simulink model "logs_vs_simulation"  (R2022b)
settings: Solver=FixedStepAuto  StartTime=0.0  StopTime=29  FixedStep=0.001  RelTol=1e-3
libraries: vrlib x2

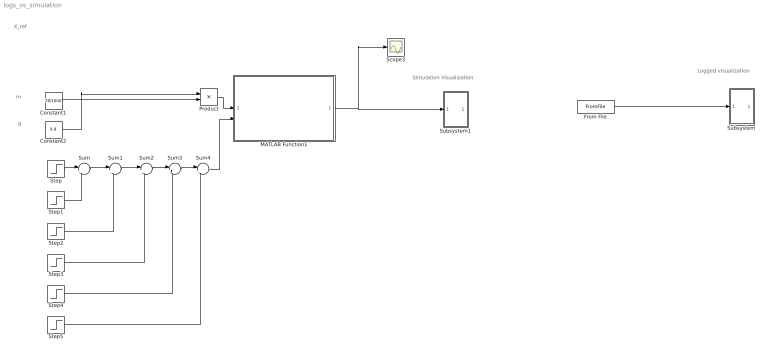
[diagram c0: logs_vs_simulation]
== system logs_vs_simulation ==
  note: Logged visualization
  note: Simulation Visualization
  note: g
  note: m
  note: X_ref
  Constant1 : Constant  Value=28/1000
  Constant2 : Constant  Value=9.8
  From File : FromFile  FileName=measured_flight_path.mat  SampleTime=0
  MATLAB Function1 : MATLAB Function  TreatAsAtomicUnit=on
  Product : Product
  Scope3 : Scope
  Step : Step  Time=2  Before=[0 0 0 0 0 0 0 0 0 0 0 0]  After=[0 0 0.66 0 0 0 0 0 0 0 0 0]  SampleTime=0
  Step1 : Step  Time=9  Before=[0 0 0 0 0 0 0 0 0 0 0 0]  After=[0.5 0 0 0 0 0 0 0 0 0 0 0]  SampleTime=0
  Step2 : Step  Time=5  Before=[0 0 0 0 0 0 0 0 0 0 0 0]  After=[0 0.6 0 0 0 0 0 0 0 0 0 0]  SampleTime=0
  Step3 : Step  Time=17  Before=[0 0 0 0 0 0 0 0 0 0 0 0]  After=[-0.5 0 0 0 0 0 0 0 0 0 0 0]  SampleTime=0
  Step4 : Step  Time=13  Before=[0 0 0 0 0 0 0 0 0 0 0 0]  After=[0 -0.6 0 0 0 0 0 0 0 0 0 0]  SampleTime=0
  Step5 : Step  Time=24  Before=[0 0 0 0 0 0 0 0 0 0 0 0]  After="[0 0 -0.66  0 0 0 0 0 0 0 0 0]"  SampleTime=0
  Subsystem : Subsystem
  Subsystem1 : Subsystem
  Sum{,1..4} (5 alike) : Sum  Inputs=|++
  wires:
  Product/1 -> MATLAB Function1/1(F_hover)
  Constant1/1 -> Product/2
  Constant2/1 -> Product/1
  MATLAB Function1/1(outputs) -> Subsystem1/1(In1), Scope3/1
  From File/1 -> Subsystem/1(In1)
  Step/1 -> Sum/1
  Step1/1 -> Sum/2
  Sum/1 -> Sum1/1
  Sum2/1 -> Sum3/1
  Sum1/1 -> Sum2/1
  Step2/1 -> Sum1/2
  Step3/1 -> Sum2/2
  Step4/1 -> Sum3/2
  Sum3/1 -> Sum4/1
  Step5/1 -> Sum4/2
  Sum4/1 -> MATLAB Function1/2(X_ref)

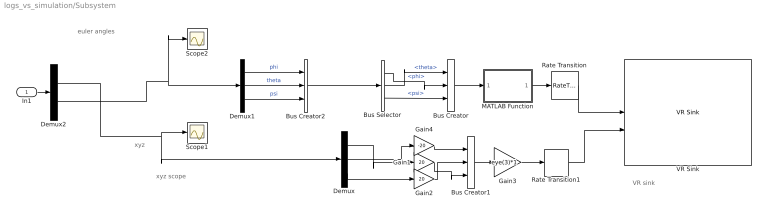
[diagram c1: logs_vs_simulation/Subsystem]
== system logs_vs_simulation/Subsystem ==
  note: VR sink
  note: xyz scope
  note: xyz
  note: euler angles
  In1 : Inport
  Bus Creator : BusCreator  Inputs=3
  Bus Creator1 : BusCreator  Inputs=3
  Bus Creator2 : BusCreator  Inputs=3
  Bus Selector : BusSelector  OutputSignals=phi,theta,psi
  Demux : Demux  Outputs=3
  Demux1 : Demux  Outputs=3
  Demux2 : Demux  Outputs=2
  Gain1 : Gain  Gain=20
  Gain2 : Gain  Gain=20
  Gain3 : Gain  Gain=eye(3)*1  Multiplication=Matrix(K*u)
  Gain4 : Gain  Gain=-20
  MATLAB Function : MATLAB Function  TreatAsAtomicUnit=on
  Rate Transition : RateTransition  OutPortSampleTime=0.06
  Rate Transition1 : RateTransition  OutPortSampleTime=0.06
  Scope1 : Scope
  Scope2 : Scope
  VR Sink : vrlib/VR Sink  InstantiateOnLoad=on  SampleTime=-1  ViewEnable=on  RemoteChange=off  RemoteView=off  FieldsWritten=Helicopter.rotation.4.1.1.double#Helicopter.translation.3.1.1.double  WorldFileName=quadrotor_world_ucart.wrl  AutoView=on  VideoDimensions=[]  AllowVariableSize=off  FigureProperties={'Position', 'Name', 'Viewpoint', 'CameraBound', 'CameraDirection', 'CameraPosition', 'CameraUpVector', 'ZoomFactor', 'Antialiasing', 'Headlight', 'Lighting', 'NavPanel', 'Sound', 'StatusBar', 'Stereo3D', 'Stereo3DCameraOffset', 'Stereo3DHIT', 'ToolBar', 'Textures', 'Transparency', 'Triad', 'Wireframe', 'NavZones', 'NavMode', 'NavSpeed', 'CaptureFileFormat', 'CaptureFileName', 'Record2DCompressMet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
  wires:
  Demux2/2 -> Scope2/1, Demux1/1
  Gain2/1 -> Bus Creator1/2
  Demux/2 -> Gain4/1
  Bus Selector/2 -> Bus Creator/1  "<theta>"
  Bus Selector/1 -> Bus Creator/2  "<phi>"
  Bus Selector/3 -> Bus Creator/3  "<psi>"
  Demux1/1 -> Bus Creator2/1  "phi"
  Bus Creator/1 -> MATLAB Function/1(u)
  Demux1/2 -> Bus Creator2/2  "theta"
  Gain4/1 -> Bus Creator1/1
  Rate Transition1/1 -> VR Sink/2
  Bus Creator2/1 -> Bus Selector/1
  Rate Transition/1 -> VR Sink/1
  Demux/3 -> Gain2/1
  Gain3/1 -> Rate Transition1/1
  Demux1/3 -> Bus Creator2/3  "psi"
  Bus Creator1/1 -> Gain3/1
  In1/1 -> Demux2/1
  MATLAB Function/1(y) -> Rate Transition/1
  Demux2/1 -> Demux/1, Scope1/1
  Demux/1 -> Gain1/1
  Gain1/1 -> Bus Creator1/3

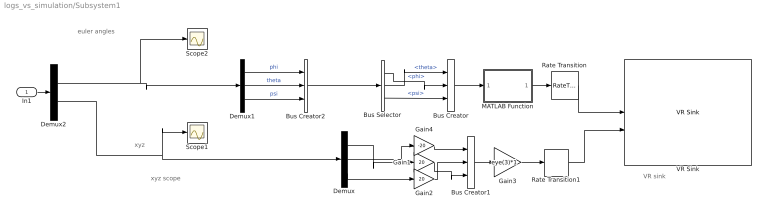
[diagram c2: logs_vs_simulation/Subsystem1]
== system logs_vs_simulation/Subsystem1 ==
  note: VR sink
  note: xyz scope
  note: xyz
  note: euler angles
  In1 : Inport
  Bus Creator : BusCreator  Inputs=3
  Bus Creator1 : BusCreator  Inputs=3
  Bus Creator2 : BusCreator  Inputs=3
  Bus Selector : BusSelector  OutputSignals=phi,theta,psi
  Demux : Demux  Outputs=3
  Demux1 : Demux  Outputs=3
  Demux2 : Demux  Outputs=2
  Gain1 : Gain  Gain=20
  Gain2 : Gain  Gain=20
  Gain3 : Gain  Gain=eye(3)*1  Multiplication=Matrix(K*u)
  Gain4 : Gain  Gain=-20
  MATLAB Function : MATLAB Function  TreatAsAtomicUnit=on
  Rate Transition : RateTransition  OutPortSampleTime=0.06
  Rate Transition1 : RateTransition  OutPortSampleTime=0.06
  Scope1 : Scope
  Scope2 : Scope
  VR Sink : vrlib/VR Sink  InstantiateOnLoad=on  SampleTime=-1  ViewEnable=on  RemoteChange=off  RemoteView=off  FieldsWritten=Helicopter.rotation.4.1.1.double#Helicopter.translation.3.1.1.double  WorldFileName=logged_playback.wrl  AutoView=on  VideoDimensions=[]  AllowVariableSize=off  FigureProperties={'Position', 'Name', 'Viewpoint', 'CameraBound', 'CameraDirection', 'CameraPosition', 'CameraUpVector', 'ZoomFactor', 'Antialiasing', 'Headlight', 'Lighting', 'NavPanel', 'Sound', 'StatusBar', 'Stereo3D', 'Stereo3DCameraOffset', 'Stereo3DHIT', 'ToolBar', 'Textures', 'Transparency', 'Triad', 'Wireframe', 'NavZones', 'NavMode', 'NavSpeed', 'CaptureFileFormat', 'CaptureFileName', 'Record2DCompressMet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
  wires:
  Gain2/1 -> Bus Creator1/2
  Demux/2 -> Gain4/1
  Bus Selector/2 -> Bus Creator/1  "<theta>"
  Bus Selector/1 -> Bus Creator/2  "<phi>"
  Bus Selector/3 -> Bus Creator/3  "<psi>"
  Demux1/1 -> Bus Creator2/1  "phi"
  Bus Creator/1 -> MATLAB Function/1(u)
  Demux1/2 -> Bus Creator2/2  "theta"
  Gain4/1 -> Bus Creator1/1
  Rate Transition1/1 -> VR Sink/2
  Bus Creator2/1 -> Bus Selector/1
  Rate Transition/1 -> VR Sink/1
  Demux/3 -> Gain2/1
  Gain3/1 -> Rate Transition1/1
  Demux1/3 -> Bus Creator2/3  "psi"
  Bus Creator1/1 -> Gain3/1
  In1/1 -> Demux2/1
  MATLAB Function/1(y) -> Rate Transition/1
  Demux/1 -> Gain1/1
  Gain1/1 -> Bus Creator1/3
  Demux2/1 -> Scope2/1, Demux1/1
  Demux2/2 -> Scope1/1, Demux/1

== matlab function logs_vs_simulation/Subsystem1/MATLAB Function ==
function y = eigenaxis_ucart(u)


if abs(u(1))< 0.0001
    u(1) = 0.0001;
end

if abs(u(2))< 0.0001
    u(2) = 0.0001;
end

if abs(u(3))< 0.0001
    u(3) = 0.0001;
end

u = [ -u(1); -u(2); u(3) ];% [Pitch, Yaw, Roll] 

C11 = cos(u(2))*cos(u(3));
C12 = cos(u(2))*sin(u(3));
C13 = -sin(u(2));
C21 = sin(u(1))*sin(u(2))*cos(u(3))-cos(u(1))*sin(u(3));
C22 = sin(u(1))*sin(u(2))*sin(u(3))+cos(u(1))*cos(u(3));
C23 = sin(u(1))*cos(u(2));
C31 = cos(u(1))*sin(u(2))*cos(u(3))+sin(u(1))*sin(u(3));
C32 = cos(u(1))*sin(u(2))*sin(u(3))-sin(u(1))*cos(u(3));
C33 = cos(u(1))*cos(u(2));
    
theta = acos(0.5*(C11+C22+C33-1));

e = [C23-C32; C31-C13; C12-C21]/(2*sin(theta));
    
y = [e; theta];

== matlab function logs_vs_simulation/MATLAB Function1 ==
function outputs = fcn(F_hover, X_ref)

coder.extrinsic('evalin', 'assignin')

Xsize = 20;

Xsize = evalin('base', 'Xsize');

X = zeros(Xsize,12);
U = zeros(1, 4);
tspan = zeros(1, 2);

X = evalin('base', 'X');
U = evalin('base', 'U');
tspan = evalin('base', 'tspan');


tspan=[tspan(2) tspan(2)+0.001];

outputs = zeros(1, 6);
[outputs, Xrot, Urot, tspanout] = compute_quad_wrapper(0.001, X, U, X_ref, F_hover, tspan);

assignin('base', 'X', Xrot);
assignin('base', 'U', Urot);
assignin('base', 'tspan', tspanout);
assignin('base', 'Xsize', size(Xrot,1))


end

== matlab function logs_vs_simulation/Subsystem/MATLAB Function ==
function y = eigenaxis_ucart(u)


if abs(u(1))< 0.0001
    u(1) = 0.0001;
end

if abs(u(2))< 0.0001
    u(2) = 0.0001;
end

if abs(u(3))< 0.0001
    u(3) = 0.0001;
end

u = [ -u(1); -u(2); u(3) ];% [Pitch, Yaw, Roll] 

C11 = cos(u(2))*cos(u(3));
C12 = cos(u(2))*sin(u(3));
C13 = -sin(u(2));
C21 = sin(u(1))*sin(u(2))*cos(u(3))-cos(u(1))*sin(u(3));
C22 = sin(u(1))*sin(u(2))*sin(u(3))+cos(u(1))*cos(u(3));
C23 = sin(u(1))*cos(u(2));
C31 = cos(u(1))*sin(u(2))*cos(u(3))+sin(u(1))*sin(u(3));
C32 = cos(u(1))*sin(u(2))*sin(u(3))-sin(u(1))*cos(u(3));
C33 = cos(u(1))*cos(u(2));
    
theta = acos(0.5*(C11+C22+C33-1));

e = [C23-C32; C31-C13; C12-C21]/(2*sin(theta));
    
y = [e; theta];
